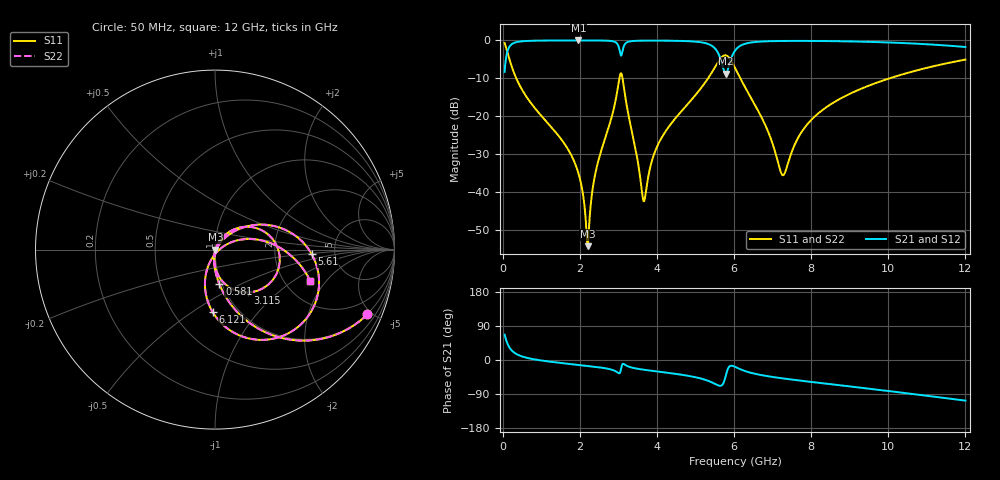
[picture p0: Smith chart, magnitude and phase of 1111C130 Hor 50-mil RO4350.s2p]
# GHz S MA R 50
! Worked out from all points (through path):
!   11951 points, 50 MHz to 12 GHz, reference 50 ohm
!   highest |S21| = -0.02 dB at 1.966 GHz (marker M1); lowest = -8.8 dB at 5.785 GHz (marker M2)
!   group delay of S21, straight-line fit = 25.4 ps
!   lowest |S11| = -54.1 dB at 2.204 GHz (marker M3), VSWR 1.00, Z = 50.2 - j0.0557 ohm
!   |S11| at or under -10 dB: 353.5 MHz to 3.027 GHz (2.674 GHz wide, 158 % of centre); 3.108 GHz to 5.325 GHz (2.216 GHz wide, 52.6 % of centre); 6.164 GHz to 10.03 GHz (3.863 GHz wide, 47.7 % of centre)
!   |S22| runs from -54.1 to -0.7 dB; largest |S21 - S12| = 0
!   S11 on the Smith chart (normalised r, x): 50 MHz: 0.97, -4.72; 581 MHz: 0.97, -0.39; 3.115 GHz: 1.26, -0.66; 5.61 GHz: 3.32, -0.23; 6.121 GHz: 0.77, -0.61; 12 GHz: 2.74, -1.40
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0.05  0.9228 -23.0  0.385 67.0  0.385 67.0  0.9228 -23.0
0.243  0.4394 -65.6  0.8978 24.3  0.8978 24.3  0.4394 -65.6
0.581  0.1931 -82.8  0.9804 7.0  0.9804 7.0  0.1931 -82.8
1.966  0.01776 -97.9  0.9982 -12.9  0.9982 -12.9  0.01776 -97.9
2.042  0.01237 -96.1  0.9981 -13.8  0.9981 -13.8  0.01237 -96.1
2.204  0.001963 -16.4  0.9979 -15.6  0.9979 -15.6  0.001963 -16.4
2.442  0.02176 63.8  0.9967 -18.5  0.9967 -18.5  0.02176 63.8
2.969  0.2103 37.2  0.9066 -32.3  0.9066 -32.3  0.2103 37.2
3.115  0.3017 -52.3  0.7549 -10.3  0.7549 -10.3  0.3017 -52.3
3.239  0.1206 -86.2  0.952 -16.3  0.952 -16.3  0.1206 -86.2
3.65  0.007785 -31.5  0.992 -25.5  0.992 -25.5  0.007785 -31.5
4.034  0.04311 51.3  0.9928 -30.6  0.9928 -30.6  0.04311 51.3
5.074  0.2123 36.8  0.9549 -47.2  0.9549 -47.2  0.2123 36.8
5.61  0.5392 -2.7  0.6443 -67.7  0.6443 -67.7  0.5392 -2.7
5.785  0.6368 -38.3  0.3633 -41.6  0.3633 -41.6  0.6368 -38.3
6.025  0.4347 -82.3  0.7318 -17.9  0.7318 -17.9  0.4347 -82.3
6.121  0.3487 -92.1  0.823 -22.5  0.823 -22.5  0.3487 -92.1
6.828  0.07343 -112.0  0.9722 -42.0  0.9722 -42.0  0.07343 -112.0
7.256  0.01689 -49.5  0.9827 -48.4  0.9827 -48.4  0.01689 -49.5
8.017  0.09146 24.5  0.9836 -58.1  0.9836 -58.1  0.09146 24.5
10.009  0.3141 6.4  0.9394 -81.9  0.9394 -81.9  0.3141 6.4
12  0.559 -18.2  0.8188 -107.2  0.8188 -107.2  0.559 -18.2
